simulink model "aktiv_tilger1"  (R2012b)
settings: Solver=ode45  StartTime=0.0  StopTime=10.0  RelTol=1e-3
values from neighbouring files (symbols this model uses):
  c1 = 20    [aktiv_tilger_1.m]    (also in aktiv_tilger_12.m; aktiv_tilger_2.m = 1; aktiv_tilger_3.m; aktiv_tilger_31.m)
  c2 = 10    [aktiv_tilger_1.m]    (also in aktiv_tilger_12.m; aktiv_tilger_3.m; aktiv_tilger_31.m; beobachter_1.m = 0.5)
  D = 0    [aktiv_tilger_1.m]    (also in aktiv_tilger_12.m; aktiv_tilger_3.m = 2000; aktiv_tilger_31.m; beobachter_1.m)
  Fe1 = 0.5    [aktiv_tilger_1.m]    (also in aktiv_tilger_12.m)
  fsig = 0.01    [aktiv_tilger_1.m]    (also in aktiv_tilger_12.m = 0.1; aktiv_tilger_2.m = 2; aktiv_tilger_3.m = 0.1; diff_filter_1.m = 1)
  I = 2000    [aktiv_tilger_1.m]    (also in aktiv_tilger_12.m; aktiv_tilger_3.m = 0; aktiv_tilger_31.m = 0; fuellstnd_2.m = 0.0225)
  k1 = 100    [aktiv_tilger_1.m]    (also in aktiv_tilger_12.m; aktiv_tilger_2.m = 5; aktiv_tilger_3.m; aktiv_tilger_31.m)
  k2 = 10    [aktiv_tilger_1.m]    (also in aktiv_tilger_12.m; aktiv_tilger_2.m = 10,      c2 = 10; aktiv_tilger_3.m; aktiv_tilger_31.m)
  m1 = 200    [aktiv_tilger_1.m]    (also in aktiv_tilger_12.m; aktiv_tilger_2.m = 100; aktiv_tilger_3.m; aktiv_tilger_31.m)
  m2 = 1    [aktiv_tilger_1.m]    (also in aktiv_tilger_12.m; aktiv_tilger_2.m = 5; aktiv_tilger_3.m; aktiv_tilger_31.m)
  P = 0    [aktiv_tilger_1.m]    (also in aktiv_tilger_12.m; aktiv_tilger_3.m; aktiv_tilger_31.m; fuellstnd_2.m = 0.09)
libraries: simulink x1

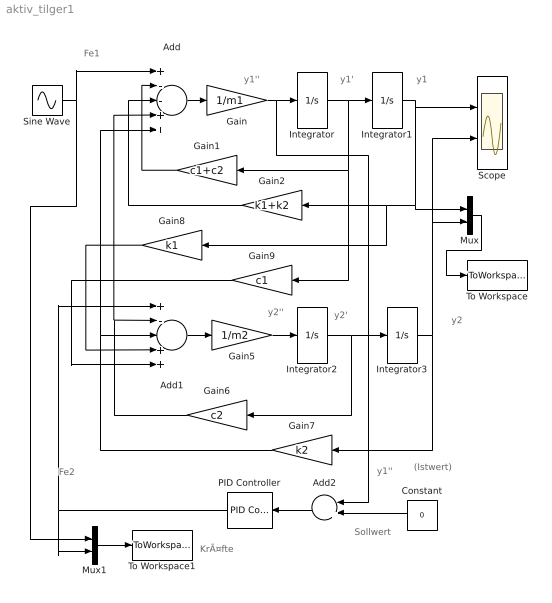
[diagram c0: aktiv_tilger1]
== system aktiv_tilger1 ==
  note: KrÃ¤fte
  note: (Istwert)
  note: Sollwert
  note: y1''
  note: Fe2
  note: Fe1
  note: y2
  note: y2'
  note: y2''
  note: y1''
  note: y1
  note: y1'
  Add : Sum  Inputs=+--++
  Add1 : Sum  Inputs=+--++
  Add2 : Sum  Inputs=-+
  Constant : Constant  Value=0
  Gain : Gain  Gain=1/m1
  Gain1 : Gain  Gain=c1+c2
  Gain2 : Gain  Gain=k1+k2
  Gain5 : Gain  Gain=1/m2
  Gain6 : Gain  Gain=c2
  Gain7 : Gain  Gain=k2
  Gain8 : Gain  Gain=k1
  Gain9 : Gain  Gain=c1
  Integrator{,1..3} (4 alike) : Integrator
  Mux : Mux  Inputs=2
  Mux1 : Mux  Inputs=2
  PID Controller : simulink/Continuous/PID Controller  Controller=PID  TimeDomain=Continuous-time  SampleTime=1  IntegratorMethod=Forward Euler  FilterMethod=Forward Euler  Form=Parallel  P=P  I=I  D=D  N=100  InitialConditionSource=internal  InitialConditionForIntegrator=0  InitialConditionForFilter=0  ExternalReset=none  LimitOutput=off  UpperSaturationLimit=inf  LowerSaturationLimit=-inf  LinearizeAsGain=on  AntiWindupMode=none  Kb=1  TrackingMode=off  Kt=1  PParamMin=[]  PParamMax=[]  IParamMin=[]  IParamMax=[]  DParamMin=[]  DParamMax=[]  NParamMin=[]  NParamMax=[]  KbParamMin=[]  KbParamMax=[]  KtParamMin=[]  KtParamMax=[]  POutMin=[]  POutMax=[]  IOutMin=[]  IOutMax=[]  DOutMin=[]  DOutMax=[]  NOutMin=[]  NOutMax=[]  KbOutMin=[]  KbOutMax=[]  KtOutMin=[]  KtOutMax=[]  IntegratorOutMin=[]  IntegratorOutMax=[]  FilterOutMin=[]  FilterOutMax=[]  SumOutMin=[]  SumOutMax=[]  SumI1OutMin=[]  SumI1OutMax=[]  SumI2OutMin=[]  SumI2OutMax=[]  SumI3OutMin=[]  SumI3OutMax=[]  SumDOutMin=[]  SumDOutMax=[]  SaturationOutMin=[]  SaturationOutMax=[]  IntegratorContinuousStateAttributes=''  IntegratorStateMustResolveToSignalObject=off  IntegratorRTWStateStorageClass=Auto  FilterContinuousStateAttributes=''  FilterStateMustResolveToSignalObject=off  FilterRTWStateStorageClass=Auto
  Scope : Scope  NumInputPorts=2
  Sine Wave : Sin  Amplitude=Fe1  Frequency=2*pi*fsig  SampleTime=0
  To Workspace : ToWorkspace  VariableName=y  SampleTime=-1  SaveFormat=Structure With Time
  To Workspace1 : ToWorkspace  VariableName=f  SampleTime=-1  SaveFormat=Structure With Time
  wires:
  Add/1 -> Gain/1
  Gain/1 -> Add2/1, Integrator/1
  Sine Wave/1 -> Add/1, Mux1/1
  Gain1/1 -> Add/2
  Gain2/1 -> Add/3
  Integrator1/1 -> Mux/1, Gain8/1, Gain2/1, Scope/1
  Gain6/1 -> Add1/2, Add/4
  Add1/1 -> Gain5/1
  Gain5/1 -> Integrator2/1
  Integrator2/1 -> Gain6/1, Integrator3/1
  Gain7/1 -> Add/5, Add1/3
  Integrator3/1 -> Gain7/1, Mux/2, Scope/2
  Gain8/1 -> Add1/4
  Gain9/1 -> Add1/5
  PID Controller/1 -> Mux1/2, Add1/1
  Integrator/1 -> Gain9/1, Gain1/1, Integrator1/1
  Mux/1 -> To Workspace/1
  Add2/1 -> PID Controller/1
  Constant/1 -> Add2/2
  Mux1/1 -> To Workspace1/1
